TYPE "StrOPDStdRx"
VERSION : 0.1


  STRUCT
   Sts_O24 : BOOL ;	//O24
   Sts_O25 : BOOL ;	//O25
   Sts_O26 : BOOL ;	//O26
   Sts_O27 : BOOL ;	//O27
   Sts_O28 : BOOL ;	//O28
   Sts_O29 : BOOL ;	//O29
   Sts_O30 : BOOL ;	//O30
   Sts_O31 : BOOL ;	//O31
   Sts_SPEED_REACHED : BOOL ;	//O16 Speed reached (absolute value higher than P47)
   Sts_POWER_ELEC_CARD : BOOL ;	//O17 Power electronic card not supplied
   Sts_IPP_DETECT_EXECUTED : BOOL ;	//O18 IPP Initial Pole position detection executed
   Sts_REGULATION_CARD : BOOL ;	//O19 Regulation card supplied and DSP not inreset state
   Sts_O20 : BOOL ;	//O20
   Sts_O21 : BOOL ;	//O21
   Sts_O22 : BOOL ;	//O22
   Sts_O23 : BOOL ;	//O23
   Sts_DRV_TORQUE_LIMIT : BOOL ;	//O08 Drive torque limit
   Sts_INCR_FOLLOW_ERROR : BOOL ;	//O09 Incremental following error
   Sts_POWER_SOFT_START_ACT : BOOL ;	//O10 Power Soft start active
   Sts_BRAKING_ACT : BOOL ;	//O11 Braking active
   Sts_NO_MAINS_POWER : BOOL ;	//O12 No mains power
   Sts_BUS_REGENERATION_EN : BOOL ;	//O13 Bus regeneration enabled (Support 1)
   Sts_EXCEED_MOTOR_THERMAL : BOOL ;	//O14 Motor thermal current exceeds threshold(P96)
   Sts_RADIATOR_OVERHEATING : BOOL ;	//O15 Radiator overheating (higher than P120 Threshold)
   Sts_READY : BOOL ;	//O00 Drive ready
   Sts_THERMAL_MOTOR_ALM : BOOL ;	//O01 Motor thermal alarm
   Sts_SPEED_GREATER_MIN : BOOL ;	//O02 Speed greater then minimum
   Sts_RUNNING : BOOL ;	//O03 Drive running
   Sts_CW_CCW : BOOL ;	//O04 CW/ CCW
   Sts_CURRENT_TORQUE : BOOL ;	//O05 Current/torque relais
   Sts_END_RAMP : BOOL ;	//O06 End Ramp
   Sts_DRIVE_CURRENT_LIMIT : BOOL ;	//O07 Drive current limit
   Sts_x0 : BOOL ;	//
   Sts_x1 : BOOL ;	//
   Sts_x2 : BOOL ;	//
   Sts_x3 : BOOL ;	//
   Sts_x4 : BOOL ;	//
   Sts_x5 : BOOL ;	//
   Sts_x6 : BOOL ;	//
   Sts_x7 : BOOL ;	//
   Sts_x8 : BOOL ;	//
   Sts_x9 : BOOL ;	//
   Sts_x10 : BOOL ;	//
   Sts_x11 : BOOL ;	//
   Sts_x12 : BOOL ;	//
   Sts_x13 : BOOL ;	//
   Sts_x14 : BOOL ;	//
   Sts_x15 : BOOL ;	//
   Sts_x16 : BOOL ;	//
   Sts_x17 : BOOL ;	//
   Sts_x18 : BOOL ;	//
   Sts_x19 : BOOL ;	//
   Sts_x20 : BOOL ;	//
   Sts_x21 : BOOL ;	//
   Sts_x22 : BOOL ;	//
   Sts_x23 : BOOL ;	//
   Sts_TARGET_REACHED : BOOL ;	//O32 Target Reached
   Sts_SP_ACHNOLEDGE : BOOL ;	//O33 Set Point Achnoledge
Sts_FOLLO_ERROR : BOOL ;	//O34 Following Error
Sts_HOMING_ATTAINED : BOOL ;	//O35 Homing attained
Sts_OP_REPLY_BIT0 : BOOL ;	//O36 OP Mode Reply Bit0
Sts_OP_REPLY_BIT1 : BOOL ;	//O37 OP Mode Reply Bit1
Sts_OP_REPLY_BIT2 : BOOL ;	//O38 OP Mode Reply Bit2
Sts_EN_OPERATION_REPLY : BOOL ;	//O39 Enable operation Reply
	AXIS_CURRENT_POSITION : DWORD ;	//AXIS CURRENT POSITION [Eng.Units]
   ALARMS : WORD ;
  END_STRUCT ;
END_TYPE

